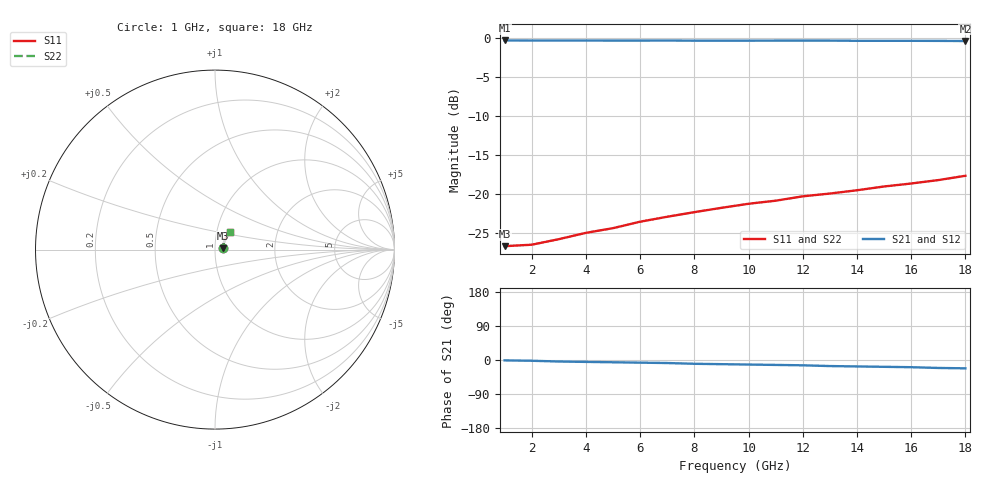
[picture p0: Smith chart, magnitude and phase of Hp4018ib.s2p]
!HPND-4018 beam lead PIN diode
!Series configuration S-parameters If=5mA.  Last updated 10/3/97
# mhz s ma r 50
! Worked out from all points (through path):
!   18 points, 1 GHz to 18 GHz, reference 50 ohm
!   highest |S21| = -0.37 dB at 1 GHz (marker M1); lowest = -0.4 dB at 18 GHz (marker M2)
!   group delay of S21, straight-line fit = 3.39 ps
!   lowest |S11| = -26.7 dB at 1 GHz (marker M3), VSWR 1.10, Z = 54.8 + j0.703 ohm
!   |S11| at or under -10 dB: start of sweep to end of sweep
!   |S22| runs from -26.7 to -17.7 dB; largest |S21 - S12| = 0
1000  0.046 8.0  0.958 -1.0  0.958 -1.0  0.046 8.0
2000  0.047 17.0  0.957 -2.0  0.957 -2.0  0.047 17.0
3000  0.051 25.0  0.957 -4.0  0.957 -4.0  0.051 25.0
4000  0.056 31.0  0.957 -5.0  0.957 -5.0  0.056 31.0
5000  0.06 36.0  0.956 -6.0  0.956 -6.0  0.06 36.0
6000  0.066 39.0  0.956 -7.0  0.956 -7.0  0.066 39.0
7000  0.071 42.0  0.957 -8.0  0.957 -8.0  0.071 42.0
8000  0.076 43.0  0.955 -10.0  0.955 -10.0  0.076 43.0
9000  0.081 45.0  0.955 -11.0  0.955 -11.0  0.081 45.0
10000  0.086 46.0  0.955 -12.0  0.955 -12.0  0.086 46.0
11000  0.09 47.0  0.956 -13.0  0.956 -13.0  0.09 47.0
12000  0.096 46.0  0.956 -14.0  0.956 -14.0  0.096 46.0
13000  0.1 47.0  0.956 -16.0  0.956 -16.0  0.1 47.0
14000  0.105 48.0  0.953 -17.0  0.953 -17.0  0.105 48.0
15000  0.111 48.0  0.953 -18.0  0.953 -18.0  0.111 48.0
16000  0.116 49.0  0.953 -19.0  0.953 -19.0  0.116 49.0
17000  0.122 48.0  0.952 -21.0  0.952 -21.0  0.122 48.0
18000  0.13 49.0  0.95 -22.0  0.95 -22.0  0.13 49.0
